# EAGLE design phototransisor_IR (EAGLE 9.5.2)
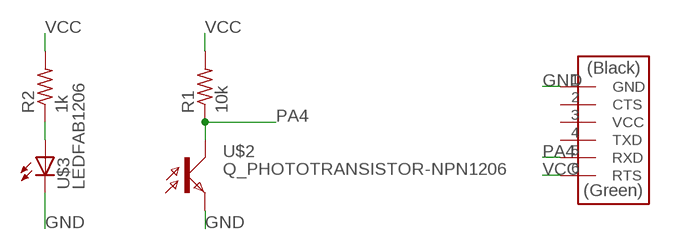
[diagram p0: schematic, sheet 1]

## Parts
R1  10k  R1206FAB  [R1206FAB]
R2  1k  R1206FAB  [R1206FAB]
U$1  CONN_06_FTDI-SMD-HEADER  [1X06SMD]
U$2  Q_PHOTOTRANSISTOR-NPN1206  [OP1206]
U$3  LEDFAB1206  [LED1206FAB]

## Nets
GND: U$1.1(GND) U$2.EMITTER(E) U$3.2(C)
N$2: R2.1 U$3.1(A)
PA4: R1.1 U$1.5(RXD) U$2.COLLECTOR(C)
VCC: R1.2 R2.2 U$1.6(RTS)
Unconnected: U$1.2(CTS) U$1.3(VCC) U$1.4(TXD)

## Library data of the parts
R1 R2 = fab:R: Resistor (US Symbol)
U$1 = fab:CONN_06_FTDI-SMD-HEADER
U$2 = fab:Q_PHOTOTRANSISTOR-NPN
U$3 = fab:LED: LED

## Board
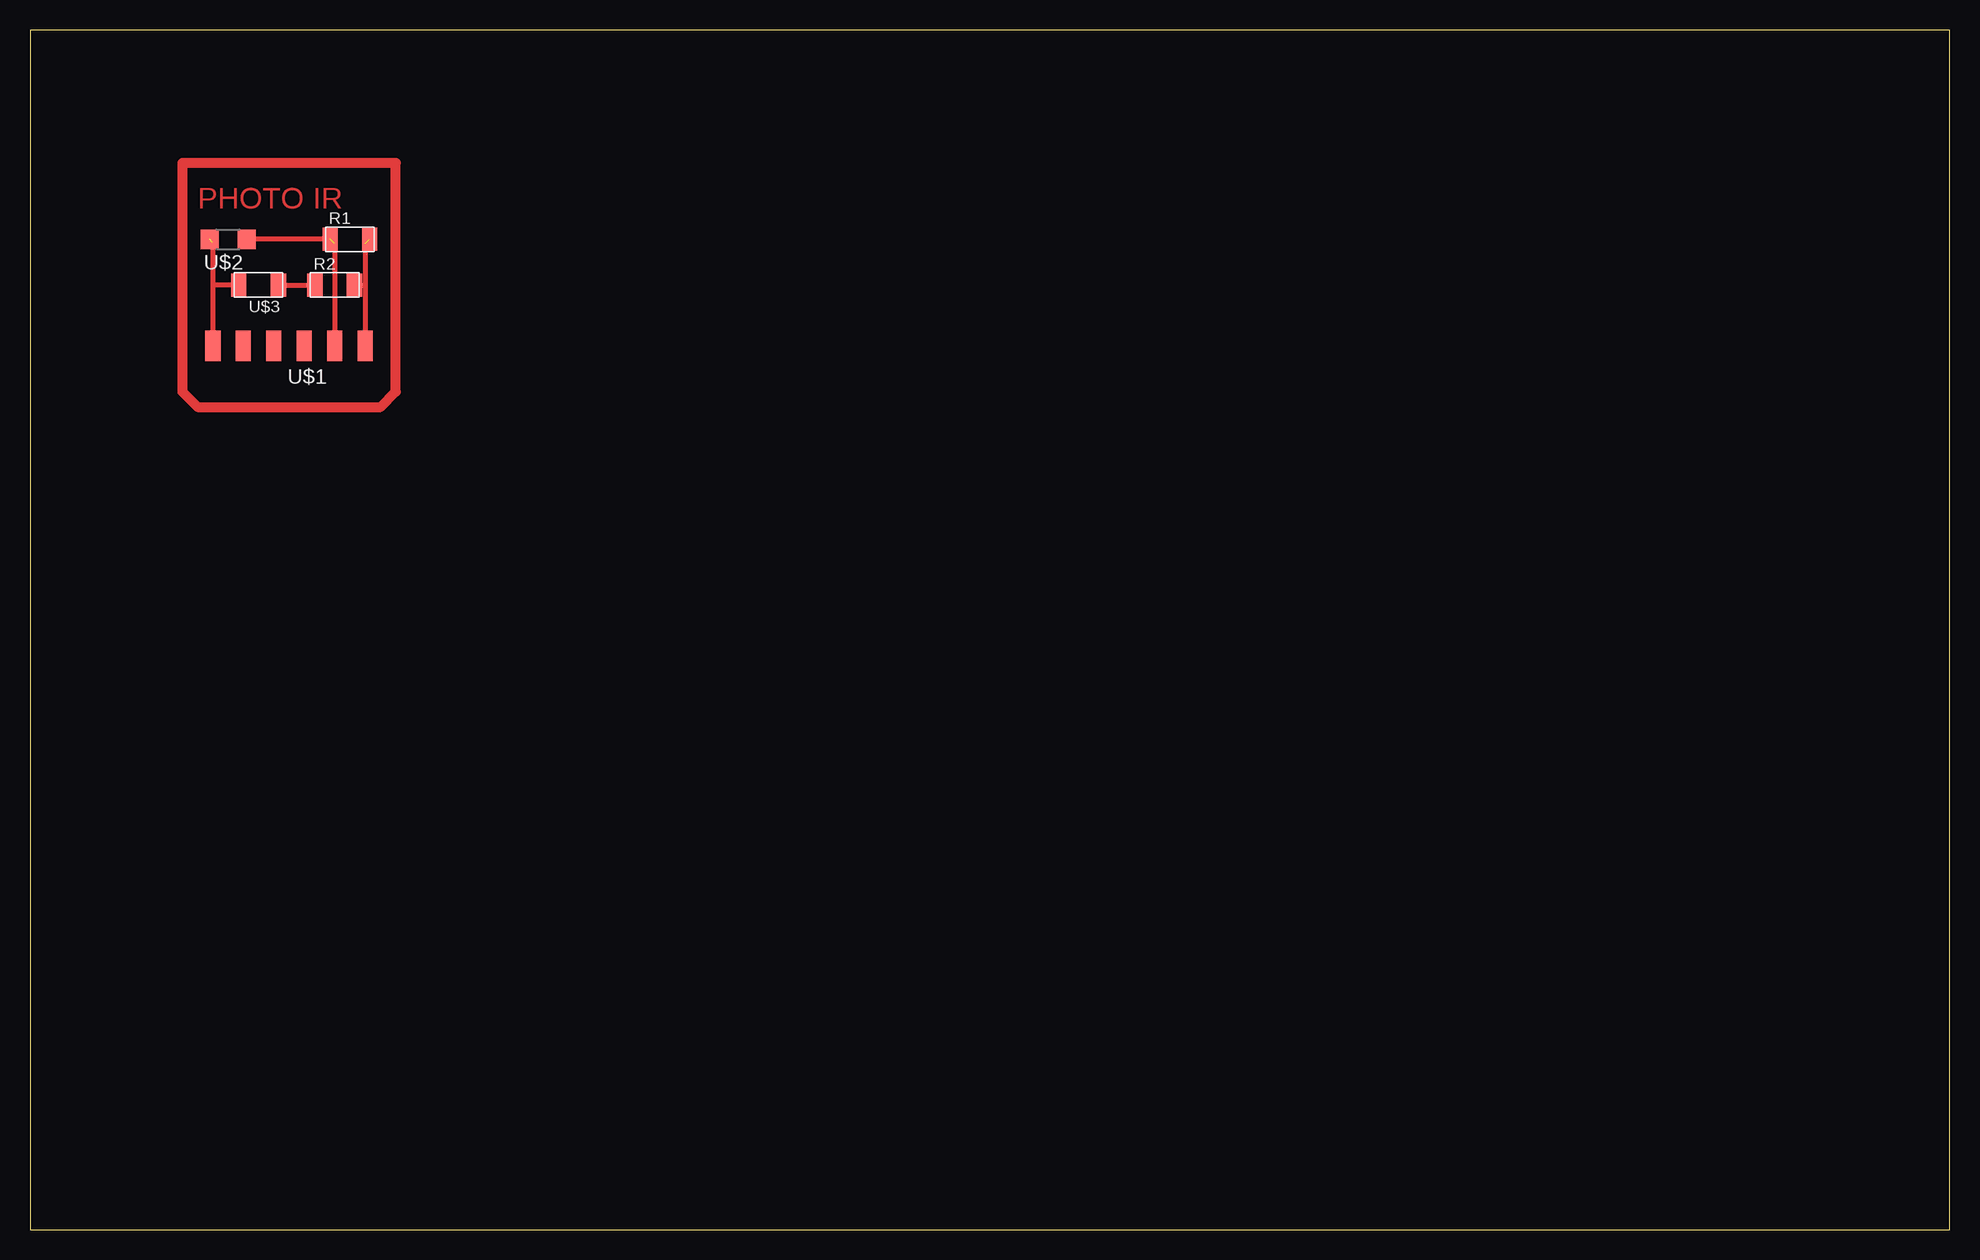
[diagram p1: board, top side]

Size 160 x 100 mm. Coordinates in mm from the lower left corner, seen from the top.
Outline: 0,0 160,0 160,100 0,100 0,0
Copper layers (1*16): Top 0.035mm / dielectric 1.5mm / Bottom 0.035mm
Design rules "default": minimum track width 6mil, minimum drill 0.35mm, track to track 6mil, track to pad 6mil, pad to pad 6mil, via to via 6mil, smd to smd 6mil, copper to edge 40mil, drill to drill 6mil, minimum pad ring 10mil, minimum via ring 8mil, stop-mask expansion 4mil, vias tented up to drill 0mil, thermal gap 10mil

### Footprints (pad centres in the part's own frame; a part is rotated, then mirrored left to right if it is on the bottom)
R1206FAB = smd 1.27 x 1.905: 1 -1.651,0; 2 1.651,0
1X06SMD = smd 2.54 x 1.27: 1 0,6.35; 2 0,3.81; 3 0,1.27; 4 0,-1.27; 5 0,-3.81; 6 0,-6.35
OP1206 = smd 1.5 x 1.6: COLLECTOR -1.55,0; EMITTER 1.55,0
LED1206FAB = smd 1.27 x 1.905: 1 -1.651,0; 2 1.651,0

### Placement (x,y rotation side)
R1  26.67,82.55 0 top
R2  25.4,78.74 0 top
U$1  21.59,73.66 90 top
U$2  16.51,82.55 180 top
U$3  19.05,78.74 180 top

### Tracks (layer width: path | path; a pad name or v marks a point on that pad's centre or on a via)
GND  (1 unrouted)
  Top 0.406: 15.24,82.27 15.24,78.74 | 15.24,78.74 U$1.1 | U$3.2 15.24,78.74
N$1
  Top 0.813: 12.7,88.9 12.7,69.85 13.97,68.58 29.21,68.58 30.48,69.85 30.48,88.9 12.7,88.9
N$2
  Top 0.406: U$3.1 R2.1
PA4  (1 unrouted)
  Top 0.406: R1.1 U$2.COLLECTOR | 25.4,82.17 U$1.5
VCC  (1 unrouted)
  Top 0.406: 27.94,82.17 27.94,78.74 | 27.94,78.74 U$1.6 | R2.2 27.94,78.74

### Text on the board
Top: PHOTO IR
